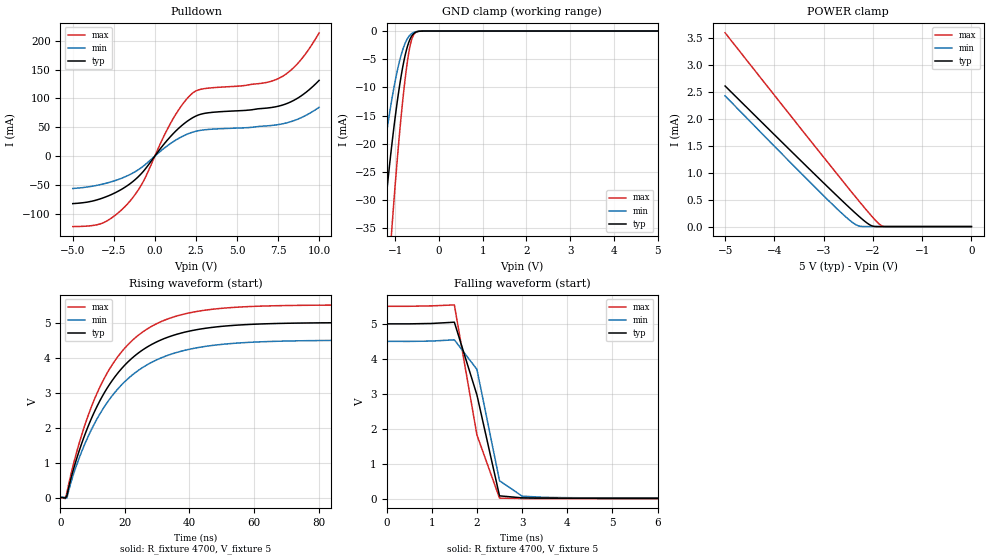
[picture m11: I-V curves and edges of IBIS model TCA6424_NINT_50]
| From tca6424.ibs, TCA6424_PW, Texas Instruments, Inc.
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[Model]   TCA6424_NINT_50
Model_type  Open_drain
Enable   Active-Low
Vref =   5
Rref =   4700
Cref =   50p
Vmeas =   2.5
| variable   typ   min   max
C_comp   2.28pF   1.90pF   2.46pF
| C_pulldown   2.95pF   2.20pF   3.72pF
| C_tri-state   2.28pF   1.90pF   2.46pF
[Temperature Range]   40   100   -40
| Ambient temperature   25   85   -40
[Voltage range]   5   4.5   5.5
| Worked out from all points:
|   slope of the pulldown table from 0 to 0.75 V, typ, clamps not added: 27.4 ohm
|   GND clamp passes 1 mA (typ) near -0.63 V on its own axis
|   POWER clamp passes 1 mA (typ) near -3.22 V on its own axis
|   rising waveform, R_fixture 4700, V_fixture 5: 20-80 % time 17.8ns typ, 18.7ns min, 16.9ns max; typ from 0.027 V to 5 V
|   falling waveform, R_fixture 4700, V_fixture 5: 20-80 % time 588ps typ, 422ps min, 547ps max; typ from 5 V to 0.027 V
[GND Clamp]
| TCA6424_NINT_50
|   Voltage   I(typ)   I(min)   I(max)
-5V       -479.6mA   -367.9mA   -640.3mA
-1.495V   -53.75mA   -35.77mA   -85.47mA
-1.45V    -49.64mA   -32.8mA    -79.5mA
-1.28V    -35.02mA   -22.38mA   -57.9mA
-1.09V    -20.8mA    -12.54mA   -36.1mA
-1.07V    -19.46mA   -11.64mA   -33.99mA
-935mV    -11.34mA   -6.326mA   -20.84mA
-800mV    -5.162mA   -2.633mA   -10.11mA
-690mV    -1.955mA   -955.9uA   -3.719mA
-585mV    -489.4uA   -264.7uA   -718.6uA
-405mV    -14.02uA   -11.66uA   -11.19uA
5V        727.1pA    2.224nA    203.5pA
[POWER Clamp]
| TCA6424_NINT_50
|   Voltage   I(typ)   I(min)   I(max)
-5V       2.602mA    2.42mA     3.587mA
-3.24V    1.021mA    787.9uA    1.559mA
-2.49V    362.7uA    132.2uA    704.6uA
-2.3V     203.7uA    16.21uA    492uA
-2.08V    42.03uA    34.33nA    251.7uA
-1.99V    6.377uA    6.423nA    157.9uA
-1.86V    68.44nA    4.325nA    39.19uA
-1.805V   10.46nA    4.167nA    9.164uA
-1.735V   2.337nA    4.002nA    409.2nA
-84.45fV  727.1pA    1.829nA    226.9pA
[Pulldown]
| TCA6424_NINT_50
|   Voltage   I(typ)   I(min)   I(max)
-5V       -82.53mA   -56.3mA    -122.4mA
-3.17V    -72.74mA   -48.6mA    -116.1mA
-1.63V    -50.43mA   -33.63mA   -81.91mA
-695mV    -26.31mA   -17.3mA    -43.63mA
465mV     17.55mA    11.31mA    29.55mA
1.13V     39.3mA     25.14mA    65.7mA
2.315V    66.7mA     41.58mA    109.6mA
3.235V    75mA       46.11mA    117.8mA
6.495V    82.46mA    51.74mA    126.2mA
7.53V     86.58mA    54.63mA    134.6mA
8.745V    101.4mA    64.52mA    162.1mA
10V       131.3mA    84.61mA    213.8mA
[Ramp]
| TCA6424_NINT_50
| variable   typ   min   max
dV/dt_r   3.00/1.78E-08   2.70/1.87E-08   3.31/1.69E-08
dV/dt_f   3.01/3.13E-10   2.71/3.95E-10   3.32/2.52E-10
R_load = 4700
[Rising Waveform]
| TCA6424_NINT_50
R_fixture =   4700
C_fixture =   0
L_fixture =   0
V_fixture =   5
V_fixture_min = 4.5
V_fixture_max = 5.5
|   Time   V(typ)   V(min)   V(max)
0s        26.77mV    37.14mV    17.43mV
1.5ns     11.55mV    26.23mV    -6.238mV
2ns       76.59mV    12.65mV    161.8mV
6ns       1.407V     1.196V     1.628V
10.5ns    2.457V     2.119V     2.81V
18.5ns    3.643V     3.184V     4.115V
30ns      4.457V     3.947V     4.974V
47ns      4.861V     4.348V     5.376V
94ns      4.997V     4.496V     5.498V
520ns     5V         4.5V       5.5V
[Falling Waveform]
| TCA6424_NINT_50
R_fixture =   4700
C_fixture =   0
L_fixture =   0
V_fixture =   5
V_fixture_min = 4.5
V_fixture_max = 5.5
|   Time   V(typ)   V(min)   V(max)
0s        5V         4.5V       5.5V
1ns       5.011V     4.509V     5.513V
1.5ns     5.046V     4.545V     5.539V
2ns       2.973V     3.701V     1.833V
2.5ns     98.49mV    529.8mV    33.55mV
3ns       41.28mV    90.26mV    22.47mV
4ns       30.22mV    46.1mV     18.82mV
9ns       26.9mV     37.42mV    17.48mV
520ns     26.77mV    37.14mV    17.43mV
